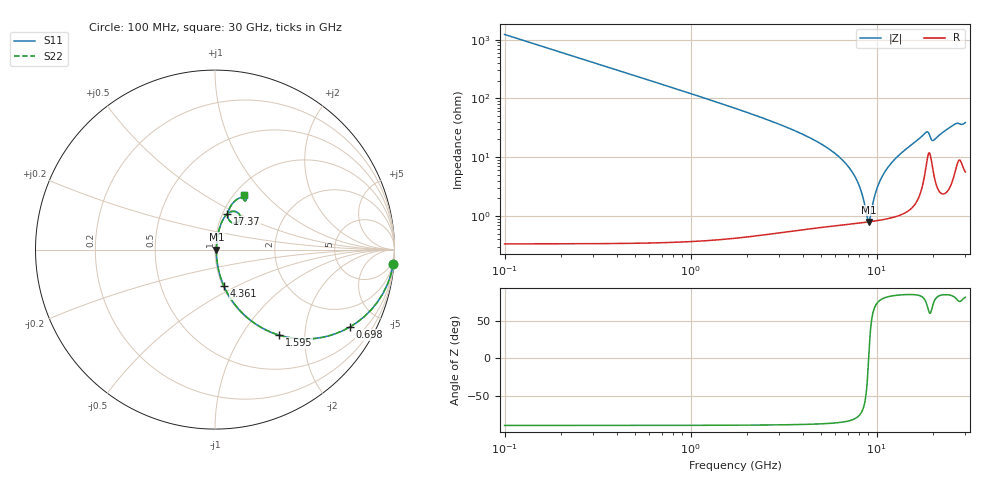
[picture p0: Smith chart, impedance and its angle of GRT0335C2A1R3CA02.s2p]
!Murata Part Number: GRT0335C2A1R3CA02
!These Parameters are Measured in Series Mode Connection
!Data Generated on Jun 19, 2026
!  o--ll--o
!Port1  Port2
!  o------o
!Operation Temp=25[degC], DC Bias Voltage=0[V]
!Freq. Start=100[MHz] Stop=30[GHz] 401[Steps]
# Hz S RI R 50
!Freq.(Hz) S11(Real) S11(Imag) S21(Real) S21(Imag) S12(Real) S12(Imag) S22(Real) S22(Imag)
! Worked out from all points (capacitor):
!   401 points, 100 MHz to 30 GHz, reference 50 ohm
!   read as one part in series: C = 1.3 pF near 249.5 MHz
!   lowest |Z| = 795 mohm at 9.07 GHz (marker M1)
!   series resonance near 9.059 GHz, so ESL is about 240 pH
!   S11 on the Smith chart (normalised r, x): 100 MHz: 1, -24; 698 MHz: 1.01, -3.49; 1.595 GHz: 1.01, -1.49; 4.361 GHz: 1.01, -0.43; 17.37 GHz: 1.05, +0.44; 30 GHz: 1.11, +0.77
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1e8  0.9933 -0.0811  0.00665 0.0811  0.00665 0.0811  0.9933 -0.0811
3.99e8  0.9034 -0.2949  0.0966 0.2949  0.0966 0.2949  0.9034 -0.2949
6.98e8  0.7519 -0.4309  0.2481 0.4309  0.2481 0.4309  0.7519 -0.4309
1.07175e9  0.5587 -0.4949  0.4413 0.4949  0.4413 0.4949  0.5587 -0.4949
1.595e9  0.3563 -0.4762  0.6437 0.4762  0.6437 0.4762  0.3563 -0.4762
2.6415e9  0.1547 -0.3559  0.8453 0.3559  0.8453 0.3559  0.1547 -0.3559
4.36075e9  0.0495 -0.2032  0.9505 0.2032  0.9505 0.2032  0.0495 -0.2032
5.10825e9  0.0318 -0.1569  0.9682 0.1569  0.9682 0.1569  0.0318 -0.1569
6.60325e9  0.0143 -0.0851  0.9857 0.0851  0.9857 0.0851  0.0143 -0.0851
7.575e9  0.00966 -0.0479  0.9903 0.0479  0.9903 0.0479  0.00966 -0.0479
8.24775e9  0.00822 -0.0251  0.9918 0.0251  0.9918 0.0251  0.00822 -0.0251
8.9205e9  0.00784 -0.00414  0.9922 0.00414  0.9922 0.00414  0.00784 -0.00414
9.07e9  0.00788 0.000321  0.9921 -0.000321  0.9921 -0.000321  0.00788 0.000321
1.01165e10  0.00918 0.0298  0.9908 -0.0298  0.9908 -0.0298  0.00918 0.0298
1.0864e10  0.0111 0.0493  0.9889 -0.0493  0.9889 -0.0493  0.0111 0.0493
1.19105e10  0.0149 0.075  0.9851 -0.075  0.9851 -0.075  0.0149 0.075
1.505e10  0.0347 0.1462  0.9653 -0.1462  0.9653 -0.1462  0.0347 0.1462
1.736725e10  0.0693 0.1996  0.9307 -0.1996  0.9307 -0.1996  0.0693 0.1996
1.871275e10  0.1316 0.2018  0.8684 -0.2018  0.8684 -0.2018  0.1316 0.2018
2.005825e10  0.085 0.1564  0.915 -0.1564  0.915 -0.1564  0.085 0.1564
2.50665e10  0.1212 0.2794  0.8788 -0.2794  0.8788 -0.2794  0.1212 0.2794
3e10  0.1635 0.304  0.8365 -0.304  0.8365 -0.304  0.1635 0.304
